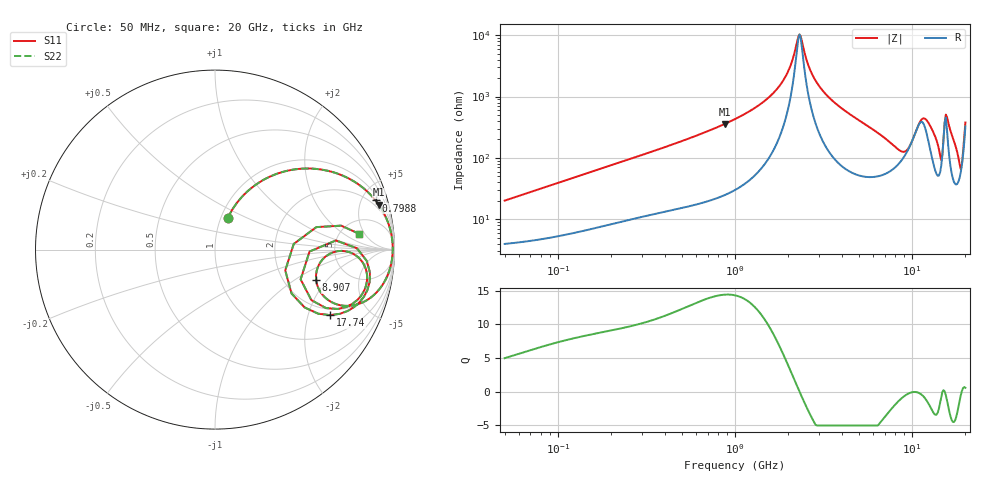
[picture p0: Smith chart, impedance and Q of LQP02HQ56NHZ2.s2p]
!Murata Part Number: LQP02HQ56NHZ2
!These Parameters are Measured in Series Mode Connection
!  o--[Z]--o
!Port1  Port2
!  o-------o
!Freq. Start=50[MHz] Stop=20[GHz], 401[Steps]
# Hz S RI R 50
!Freq.(Hz) S11(Real) S11(Imag) S21(Real) S21(Imag) S12(Real) S12(Imag) S22(Real) S22(Imag)
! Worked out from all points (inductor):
!   401 points, 50 MHz to 20 GHz, reference 50 ohm
!   read as one part in series: L = 62.5 nH near 51.52 MHz
!   highest Q = 14.4 at 873.9 MHz (marker M1), where L = 65 nH
!   self-resonance near 2.314 GHz
!   S11 on the Smith chart (normalised r, x): 50 MHz: 1.08, +0.39; 798.8 MHz: 1.45, +6.36; 8.907 GHz: 2.99, -1.54; 17.74 GHz: 1.74, -2.78; 20 GHz: 7.53, +3.82
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5e7  0.0716 0.1762  0.9284 -0.1762  0.9284 -0.1762  0.0716 0.1762
1.364002e8  0.2433 0.3724  0.7567 -0.3724  0.7567 -0.3724  0.2433 0.3724
3.721004e8  0.6458 0.4348  0.3542 -0.4348  0.3542 -0.4348  0.6458 0.4348
7.987718e8  0.8948 0.2738  0.1052 -0.2738  0.1052 -0.2738  0.8948 0.2738
8.738837e8  0.9127 0.2497  0.0873 -0.2497  0.0873 -0.2497  0.9127 0.2497
1e9  0.9352 0.2136  0.0648 -0.2136  0.0648 -0.2136  0.9352 0.2136
1.766834e9  0.9857 0.0669  0.0143 -0.0669  0.0143 -0.0669  0.9857 0.0669
2.021818e9  0.9894 0.0336  0.0106 -0.0336  0.0106 -0.0336  0.9894 0.0336
2.313601e9  0.9904 0.000217  0.00962 -0.000217  0.00962 -0.000217  0.9904 0.000217
2.728004e9  0.9878 -0.0412  0.0122 0.0412  0.0122 0.0412  0.9878 -0.0412
3.792786e9  0.9667 -0.13  0.0333 0.13  0.0333 0.13  0.9667 -0.13
7.442007e9  0.7121 -0.3123  0.2879 0.3123  0.2879 0.3123  0.7121 -0.3123
8.907419e9  0.5634 -0.1683  0.4366 0.1683  0.4366 0.1683  0.5634 -0.1683
1.019291e10  0.6833 -0.00871  0.3167 0.00871  0.3167 0.00871  0.6833 -0.00871
1.149051e10  0.8281 -0.0802  0.1719 0.0802  0.1719 0.0802  0.8281 -0.0802
1.314879e10  0.8126 -0.2588  0.1874 0.2588  0.1874 0.2588  0.8126 -0.2588
1.438523e10  0.5368 -0.2814  0.4632 0.2814  0.4632 0.2814  0.5368 -0.2814
1.504638e10  0.6731 0.0509  0.3269 -0.0509  0.3269 -0.0509  0.6731 0.0509
1.573793e10  0.8633 -0.128  0.1367 0.128  0.1367 0.128  0.8633 -0.128
1.774144e10  0.6409 -0.3652  0.3591 0.3652  0.3591 0.3652  0.6409 -0.3652
1.88369e10  0.3913 -0.1158  0.6087 0.1158  0.6087 0.1158  0.3913 -0.1158
2e10  0.8047 0.0875  0.1953 -0.0875  0.1953 -0.0875  0.8047 0.0875
